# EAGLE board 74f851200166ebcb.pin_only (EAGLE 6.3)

Size 20.32 x 16.51 mm. Coordinates in mm from the lower left corner, seen from the top.
Outline: 20.32,2.54 20.32,13.97 arc90 17.78,16.51 2.54,16.51 arc90 0,13.97 0,2.54 arc90 2.54,0 17.78,0 arc90 20.32,2.54
Copper layers (1*16): Top 0.035mm / dielectric 1.5mm / Bottom 0.035mm
Design rules "adafruit": minimum track width 8mil, minimum drill 15.5mil, track to track 8mil, track to pad 8mil, pad to pad 8mil, via to via 8mil, smd to smd 8mil, copper to edge 10mil, drill to drill 8mil, minimum pad ring 10mil, minimum via ring 8mil, stop-mask expansion 4mil, vias tented up to drill 20mil, thermal gap 10mil

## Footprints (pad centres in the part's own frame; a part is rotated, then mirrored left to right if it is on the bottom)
0805-NO = smd 1.3 x 1.5: 1 -0.95,0; 2 0.95,0
SOT23-R = smd 0.635 x 1.016: 1 -0.95,-1; 2 0.95,-1; 3 0,1
0805 = smd 1.3 x 1.5: 1 -0.95,0; 2 0.95,0
FIDUCIAL_1MM = smd 1 x 1: 1 0,0
1X04_ROUND = drill 1 pad 1.676 square: 1 -3.81,0 | drill 1 pad 1.676: 2 -1.27,0; 3 1.27,0; 4 3.81,0
MSOP8_0.65MM = smd 0.4 x 1.4: 1 -0.975,-2.2; 2 -0.325,-2.2; 3 0.325,-2.2; 4 0.975,-2.2; 5 0.975,2.2; 6 0.325,2.2; 7 -0.325,2.2; 8 -0.975,2.2
MOUNTINGHOLE_2.5_PLATED = drill 2.5 pad 3.2: P$1 0,0
TERMBLOCK_1X2-3.5MM = drill 1 pad 2.184: 1 1.8,0; 2 -1.7,0

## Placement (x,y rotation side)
C1  0.1µF  [0805-NO]  11.94,13.97 270 top
C2  0.01uF  [0805-NO]  10.16,2.79 270 top
C3  0.1uF  [0805-NO]  9.02,8.38 270 top
C4  0.01uF  [0805-NO]  9.91,13.97 270 top
D1  TLVH431  [SOT23-R]  12.74,3.38 180 top
FB1  ferrite  [0805]  15.49,12.19 270 top
FID1  FIDUCIAL""  [FIDUCIAL_1MM]  18.29,1.78 0 top
FID2  FIDUCIAL""  [FIDUCIAL_1MM]  7.82,13.43 0 top
JP1  [1X04_ROUND]  17.78,7.87 270 top
R1  100  [0805-NO]  9.14,11.18 0 top
R2  100  [0805-NO]  9.14,5.59 0 top
R3  1M  [0805-NO]  8.13,2.79 90 top
R4  1K  [0805-NO]  15.52,3.51 270 top
U1  AD8495ARMZ  [MSOP8_0.65MM]  12.7,8.38 0 top
U$8  [SYMBOL_PLUS]  5.59,13.21 0 top
U$9  [SYMBOL_MINUS]  5.59,3.3 0 top
U$10  [ADAFRUIT_2.5MM]  17.5,13.04 0 top
U$11  MOUNTINGHOLE2.5  [MOUNTINGHOLE_2.5_PLATED]  2.54,13.97 0 top
U$12  MOUNTINGHOLE2.5  [MOUNTINGHOLE_2.5_PLATED]  2.54,2.54 0 top
U$13  [ADAFRUIT_3.5MM]  15.49,12.7 90 bottom
X1  3.5mm terminal  [TERMBLOCK_1X2-3.5MM]  3.3,8.38 270 top

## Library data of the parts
C1-C4 D1 FB1 JP1 R1-R4 U1 U$8-U$10 U$13 X1 = microbuilder
FID1 FID2 U$11 U$12 = microbuilder; BOM: EXCLUDE

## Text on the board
tPlace: AD8495 | Ylw | V+ | GND | OUT | GND | Red | adafruit!
bPlace: AD8495 | Analog K-type / Thermocouple / Amplifier | V+: 2.7-18VDC | Output voltage: | T=(Vo-1.25)/5mV | Vo=T*5mV+1.25V | Temp is in °C

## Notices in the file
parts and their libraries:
microbuilder: This work is placed in the public domain, and may be freely used for commercial and non-commercial work with the following conditions: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
